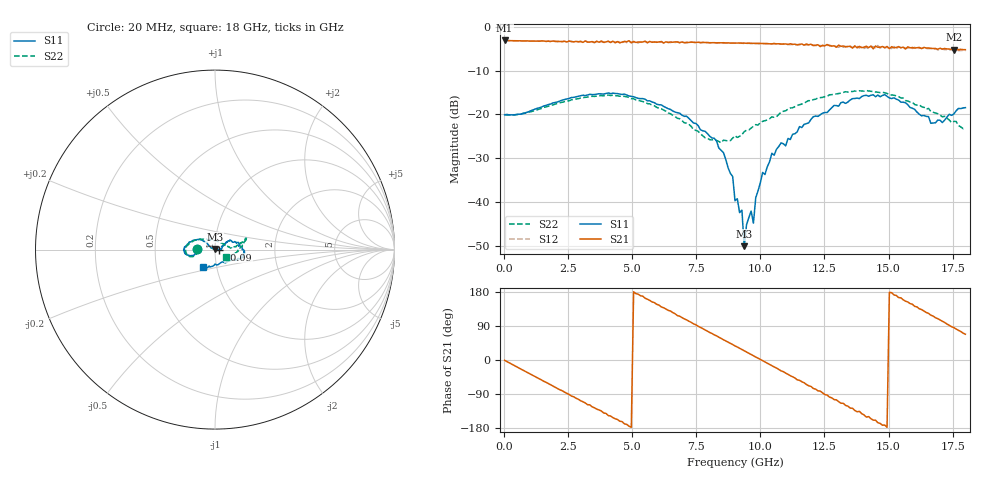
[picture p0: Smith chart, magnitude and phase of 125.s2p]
!Agilent Technologies,N5230A,US43500223,A.07.50.48
!Agilent N5230A: A.07.50.48
!Date: Thursday, January 14, 2016 17:27:54
!Correction: S11(Full 2 Port(1,2))
!S21(Full 2 Port(1,2))
!S12(Full 2 Port(1,2))
!S22(Full 2 Port(1,2))
!S2P File: Measurements: S11, S21, S12, S22:
# Hz S  dB  R 50
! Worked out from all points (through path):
!   201 points, 20 MHz to 18 GHz, reference 50 ohm
!   highest |S21| = -3.14 dB at 20 MHz (marker M1); lowest = -5.3 dB at 17.55 GHz (marker M2)
!   group delay of S21, straight-line fit = 100 ps
!   lowest |S11| = -50.1 dB at 9.37 GHz (marker M3), VSWR 1.01, Z = 49.9 + j0.301 ohm
!   |S11| at or under -10 dB: start of sweep to end of sweep
!   |S22| runs from -26.5 to -14.6 dB; largest |S21 - S12| = 0.06
!   S11 on the Smith chart (normalised r, x): 20 MHz: 0.82, +0.00; 10.09 GHz: 1.04, -0.00; 18 GHz: 0.86, -0.17
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2e7  -20.12 179.2  -3.14 -0.8  -3.16 -0.9  -20.07 179.5
1.7281e9  -17.77 -165.0  -3.31 -62.2  -3.29 -63.1  -18.14 -162.4
3.0766e9  -15.64 -171.1  -3.58 -110.1  -3.52 -110.9  -16.19 -167.5
4.6948e9  -15.38 174.9  -3.36 -168.5  -3.37 -168.8  -15.91 173.5
6.0433e9  -17.82 156.3  -3.47 145.0  -3.69 143.7  -18.61 152.8
7.212e9  -20.93 143.3  -3.59 102.3  -3.58 100.8  -22.28 129.8
8.2908e9  -26.11 143.5  -3.69 63.7  -3.69 61.7  -25.97 82.9
8.9201e9  -34.19 153.8  -3.73 40.8  -3.74 38.9  -25.45 42.8
9.01e9  -39.73 161.7  -3.75 37.1  -3.75 35.5  -24.90 37.0
9.2797e9  -41.88 96.7  -3.76 27.7  -3.78 25.7  -24.66 26.5
9.3696e9  -50.09 105.3  -3.74 24.4  -3.82 22.7  -23.94 25.8
9.6393e9  -42.09 23.6  -3.80 14.5  -3.83 12.7  -23.14 16.7
9.7292e9  -44.85 9.5  -3.79 11.4  -3.84 9.7  -22.73 14.6
9.8191e9  -39.03 -28.1  -3.81 7.9  -3.82 6.1  -22.35 12.0
1.00888e10  -33.26 -0.1  -3.83 -1.7  -3.83 -3.7  -21.61 8.0
1.20666e10  -20.54 30.4  -4.33 -75.2  -4.13 -75.9  -16.65 15.1
1.32353e10  -17.23 13.0  -4.41 -114.2  -4.67 -118.3  -15.01 18.2
1.41343e10  -15.66 -4.7  -4.46 -150.7  -4.71 -149.9  -14.58 19.7
1.50333e10  -16.27 -15.9  -5.00 178.6  -4.98 175.7  -15.53 14.8
1.66515e10  -22.04 -59.4  -4.95 118.2  -4.97 114.8  -19.36 -14.6
1.75505e10  -19.90 -109.5  -5.27 85.4  -5.46 81.4  -21.62 -25.0
1.8e10  -18.48 -125.3  -5.25 68.0  -5.47 64.7  -22.99 -34.0
